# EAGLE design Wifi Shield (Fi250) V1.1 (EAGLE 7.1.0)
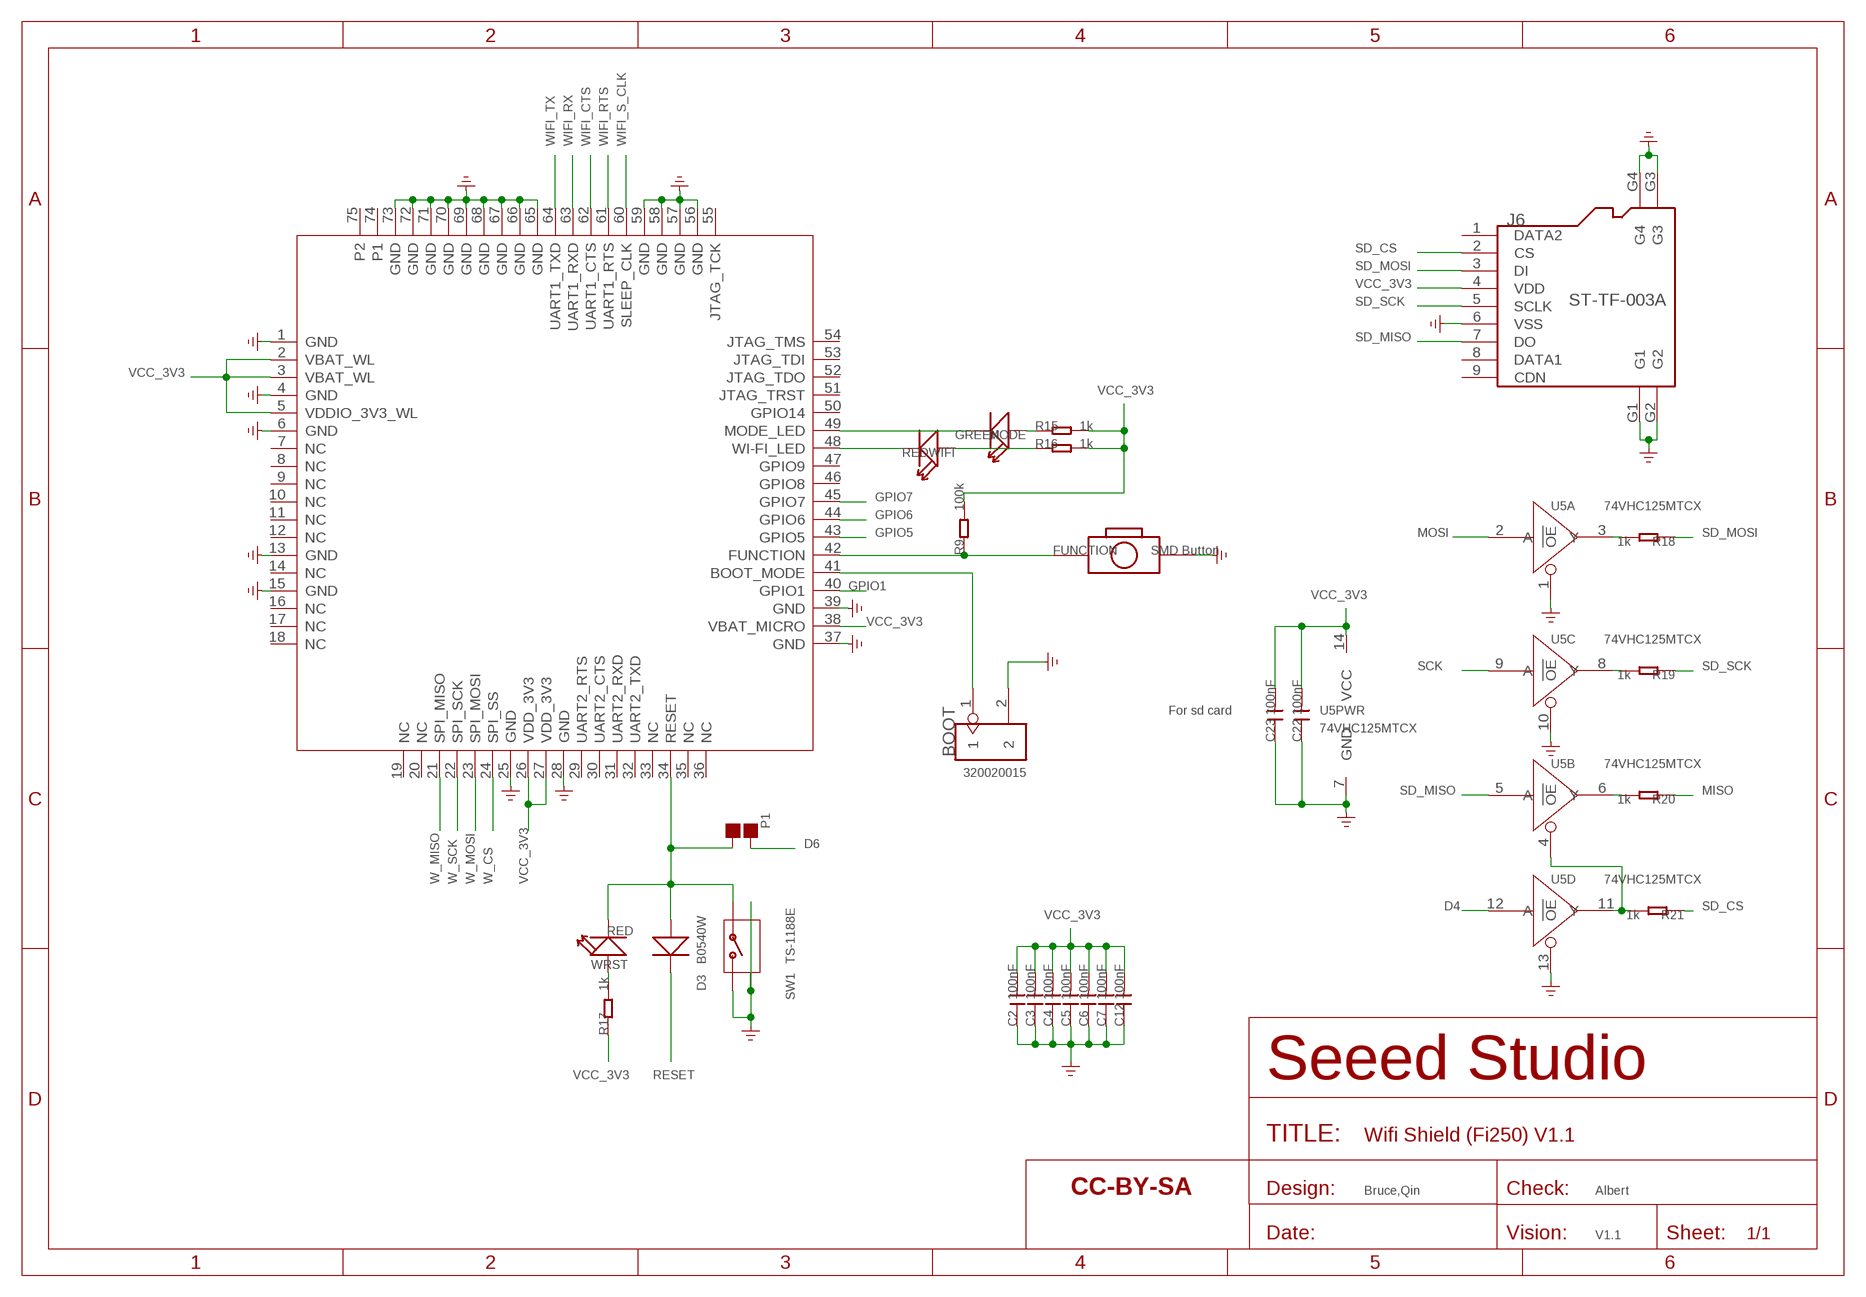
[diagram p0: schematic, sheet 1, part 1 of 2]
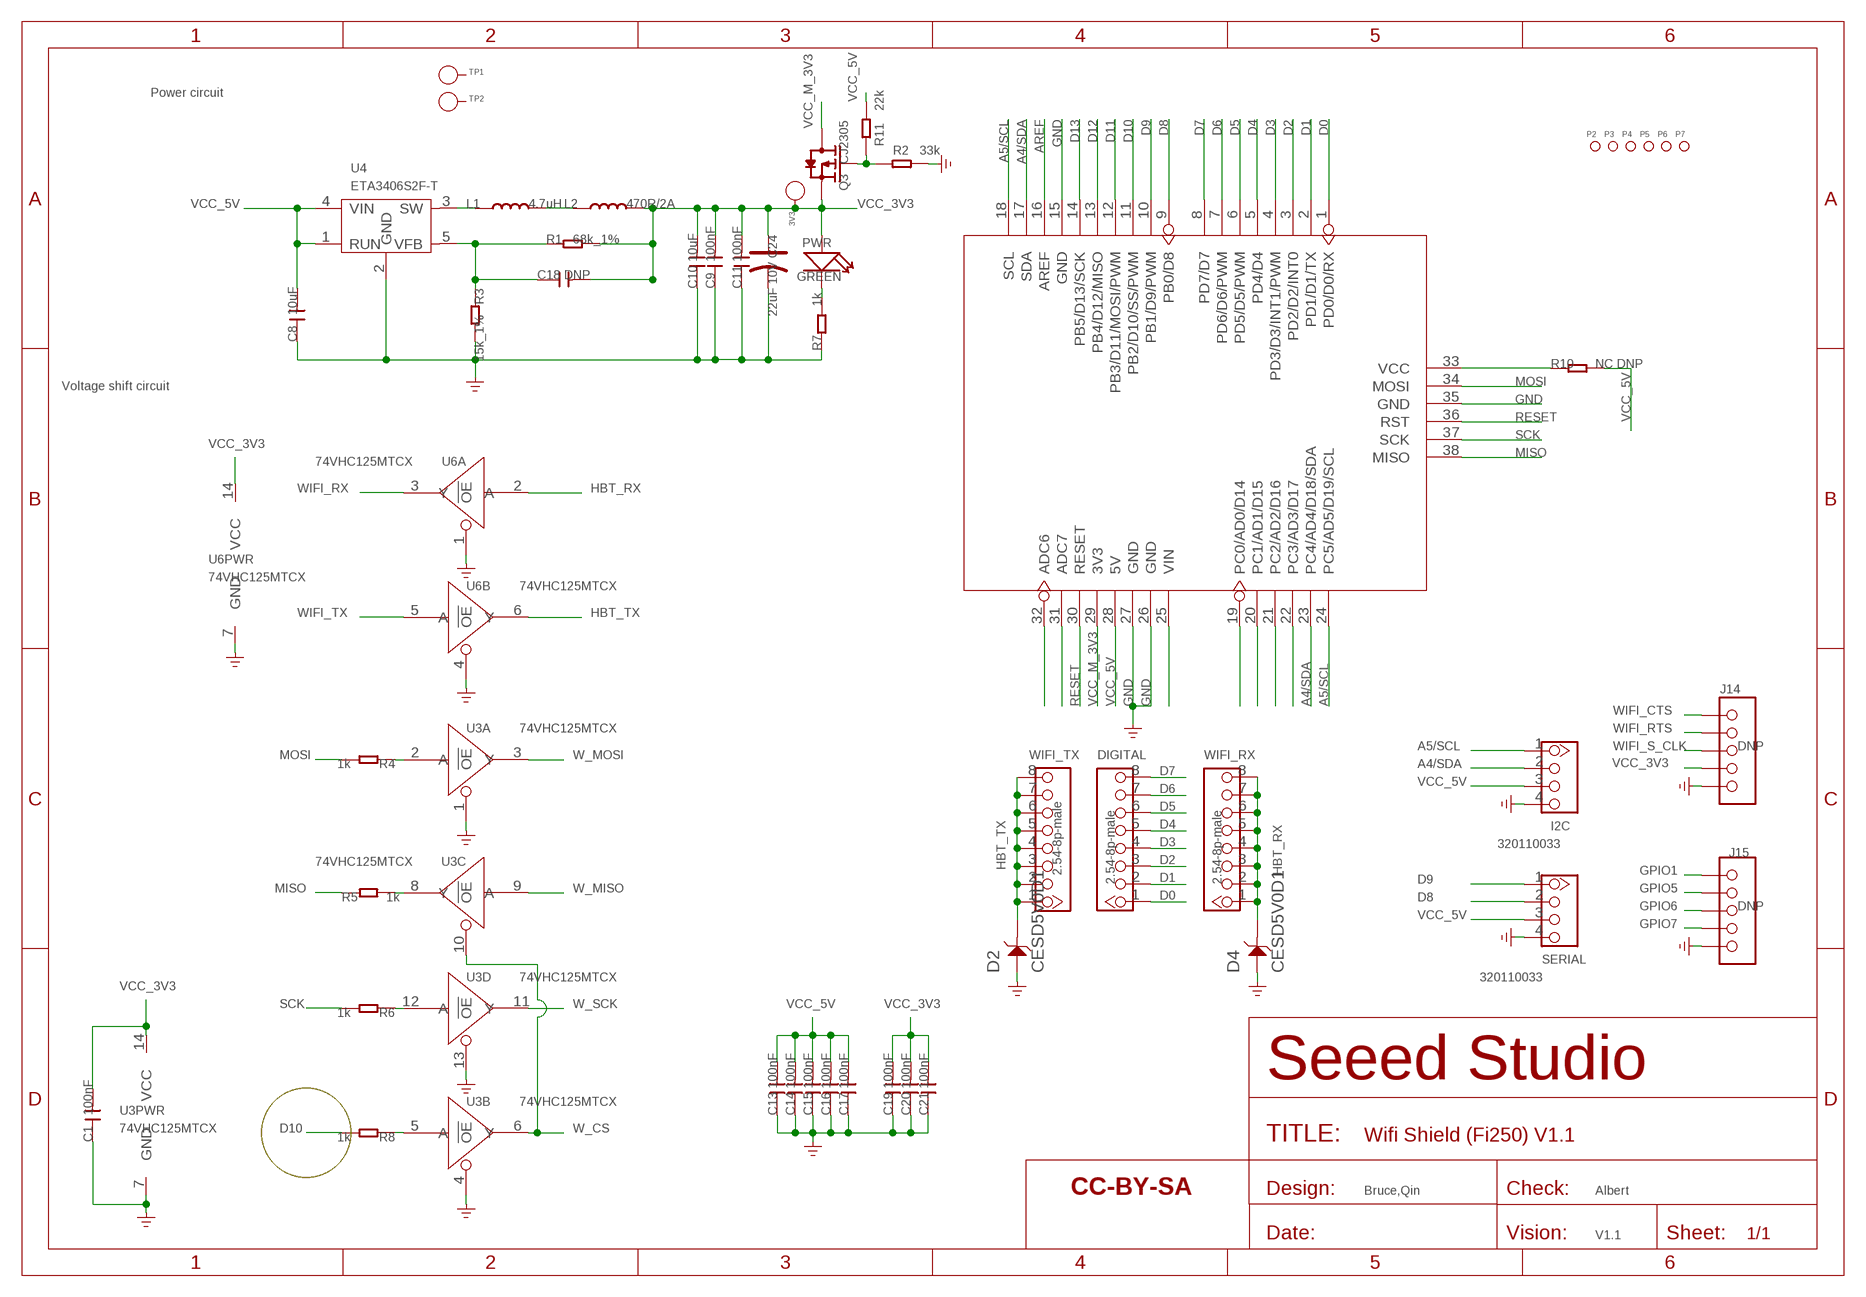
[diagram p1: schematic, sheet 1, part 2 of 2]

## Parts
3V3  PAD-TEST-POINT'4545'  [TP_4545]
BOOT  320020015  HEADER-2P-65/35MIL  [2P-2.54-65/35MIL]
C1  100nF  C-0603  [C0603]
C2  100nF  C-0603  [C0603]
C3  100nF  C-0603  [C0603]
C4  100nF  C-0603  [C0603]
C5  100nF  C-0603  [C0603]
C6  100nF  C-0603  [C0603]
C7  100nF  C-0603  [C0603]
C8  10uF  C-0805  [C0805]
C9  100nF  C-0603  [C0603]
C10  10uF  C-0805  [C0805]
C11  100nF  C-0603  [C0603]
C12  100nF  C-0603  [C0603]
C13  100nF  C-0603  [C0603]
C14  100nF  C-0603  [C0603]
C15  100nF  C-0603  [C0603]
C16  100nF  C-0603  [C0603]
C17  100nF  C-0603  [C0603]
C18  DNP  C-0603  [C0603]
C19  100nF  C-0603  [C0603]
C20  100nF  C-0603  [C0603]
C21  100nF  C-0603  [C0603]
C22  100nF  C-0603  [C0603]
C23  100nF  C-0603  [C0603]
C24  22uF 10V  CAP-AVX-A  [AVX-A]
D2  CESD5V0D1  D-ESD-2P'CESD5V0D1'  [SOD123-2.7X1.6]
D3  B0540W  D'1206'  [SOD123]
D4  CESD5V0D1  D-ESD-2P'CESD5V0D1'  [SOD123-2.7X1.6]
DIGITAL  2.54-8p-male  HEADER-8P-2.54  [8P-2.54]
FUNCTION  SMD Button  BUTTON-2P-SMD  [2P-SMD-6.1X3.81]
I2C  320110033  TWIG-4P-2.0-2.0  [4P-2.0]
J6  ST-TF-003A  HOLDER-MICROSD-9P  [9P-SMD-W/-RING]
J14  DNP  HEADER-5P-2.54  [5P-2.54]
J15  DNP  HEADER-5P-2.54  [5P-2.54]
L1  4.7uH  LSPD3D16-4R7M  [L0420]
L2  470R/2A  L'0805'  [L0805]
MODE  GREEN  LED'0603'  [LED-0603]
P1  DNP  PAD-JUMPER-2P  [2P-SMD-1.78X1.27]
P2  PAD-MARK  [ROUND-MARK-1.0]
P3  PAD-MARK  [ROUND-MARK-1.0]
P4  PAD-MARK  [ROUND-MARK-1.0]
P5  PAD-MARK  [ROUND-MARK-1.0]
P6  PAD-MARK  [ROUND-MARK-1.0]
P7  PAD-MARK  [ROUND-MARK-1.0]
PWR  GREEN  LED'0603'  [LED-0603]
Q3  CJ2305  MOSFET-P'SI2323CDS/SI2305DS<BR>'  [SOT23]
R1  68k_1%  R-0603  [R0603]
R2  33k  R-0603  [R0603]
R3  15k_1%  R-0603  [R0603]
R4  1k  R-0603  [R0603]
R5  1k  R-0603  [R0603]
R6  1k  R-0603  [R0603]
R7  1k  R-0603  [R0603]
R8  1k  R-0603  [R0603]
R9  100k  R-0603  [R0603]
R10  NC DNP  R-0603  [R0603]
R11  22k  R-0603  [R0603]
R15  1k  R-0603  [R0603]
R16  1k  R-0603  [R0603]
R17  1k  R-0603  [R0603]
R18  1k  R-0603  [R0603]
R19  1k  R-0603  [R0603]
R20  1k  R-0603  [R0603]
R21  1k  R-0603  [R0603]
SERIAL  320110033  TWIG-4P-2.0-2.0  [4P-2.0]
SW1  TS-1188E  BUTTON-4P-REINFORCE'TS-1188E'  [4P-SMD-7X3.5X3.5H]
TP1  PAD-TEST-POINT'4545'  [TP_4545]
TP2  PAD-TEST-POINT'4545'  [TP_4545]
U1  WIZFI250  [73P-28X20MM]
U2  206000005  ARDUINO-38P'WITH-SILK'  [ARDUINO-DIM-WITH-SILK]
U3  74VHC125MTCX  74VHCT125PW  [TSSOP14]
U4  ETA3406S2F-T  TD6810'TSOT23-5'  [SOT23-5]
U5  74VHC125MTCX  74VHC125PW  [TSSOP14]
U6  74VHC125MTCX  74VHC125PW  [TSSOP14]
U$1  SEEEDSTUDIO-OPEN-SCH-FRAME  [SEEEDSTUDIO-PCB-FRAME]
U$2  SEEEDSTUDIO-OPEN-SCH-FRAME  [SEEEDSTUDIO-PCB-FRAME]
WIFI  RED  LED'0603'  [LED-0603]
WIFI_RX  2.54-8p-male  HEADER-8P-2.54  [8P-2.54]
WIFI_TX  2.54-8p-male  HEADER-8P-2.54  [8P-2.54]
WRST  RED  LED'0603'  [LED-0603]

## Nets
A4/SDA: I2C.2 U2.17(SDA) U2.23(PC4/AD4/D18/SDA)
A5/SCL: I2C.1 U2.18(SCL) U2.24(PC5/AD5/D19/SCL)
AREF: U2.16(AREF)
D0: DIGITAL.1 U2.1(PD0/D0/RX)
D1: DIGITAL.2 U2.2(PD1/D1/TX)
D2: DIGITAL.3 U2.3(PD2/D2/INT0)
D3: DIGITAL.4 U2.4(PD3/D3/INT1/PWM)
D4: DIGITAL.5 U2.5(PD4/D4) U5.12(D:A)
D5: DIGITAL.6 U2.6(PD5/D5/PWM)
D6: DIGITAL.7 P1.2 U2.7(PD6/D6/PWM)
D7: DIGITAL.8 U2.8(PD7/D7)
D8: SERIAL.2 U2.9(PB0/D8)
D9: SERIAL.1 U2.10(PB1/D9/PWM)
D10: R8.2 U2.11(PB2/D10/SS/PWM)
D11: U2.12(PB3/D11/MOSI/PWM)
D12: U2.13(PB4/D12/MISO)
D13: U2.14(PB5/D13/SCK)
GND: BOOT.2 C1.1 C2.1 C3.1 C4.1 C5.1 C6.1 C7.1 C8.1 C9.1 C10.1 C11.1 C12.1 C13.1 C14.1 C15.1 C16.1 C17.1 C19.1 C20.1 C21.1 C22.1 C23.1 C24.- D2.1 D4.1 FUNCTION.P$2 I2C.4 J6.6(VSS) J6.G1 J6.G2 J6.G3 J6.G4 J14.5 J15.5 R2.1 R3.2 R7.1 SERIAL.4 SW1.2 SW1.S1 SW1.S2 U1.1(GND) U1.4(GND) U1.6(GND) U1.13(GND) U1.15(GND) U1.25(GND) U1.28(GND) U1.37(GND) U1.39(GND) U1.56(GND) U1.57(GND) U1.58(GND) U1.59(GND) U1.65(GND) U1.66(GND) U1.67(GND) U1.68(GND) U1.69(GND) U1.70(GND) U1.71(GND) U1.72(GND) U1.73(GND) U2.15(GND) U2.26(GND) U2.27(GND) U2.35(GND) U3.1(A:!OE) U3.4(B:!OE) U3.7(PWR:GND) U3.13(D:!OE) U4.2(GND) U5.1(A:!OE) U5.7(PWR:GND) U5.10(C:!OE) U5.13(D:!OE) U6.1(A:!OE) U6.4(B:!OE) U6.7(PWR:GND)
GPIO1: J15.1 U1.40(GPIO1)
GPIO5: J15.2 U1.43(GPIO5)
GPIO6: J15.3 U1.44(GPIO6)
GPIO7: J15.4 U1.45(GPIO7)
HBT_RX: D4.2 U6.2(A:A) WIFI_RX.1 WIFI_RX.2 WIFI_RX.3 WIFI_RX.4 WIFI_RX.5 WIFI_RX.6 WIFI_RX.7 WIFI_RX.8
HBT_TX: D2.2 U6.6(B:Y) WIFI_TX.1 WIFI_TX.2 WIFI_TX.3 WIFI_TX.4 WIFI_TX.5 WIFI_TX.6 WIFI_TX.7 WIFI_TX.8
MISO: R5.1 R20.1 U2.38(MISO)
MOSI: R4.2 U2.34(MOSI) U5.2(A:A)
N$1: R10.1 U2.33(VCC)
N$2: BOOT.1 U1.41(BOOT_MODE)
N$3: R4.1 U3.2(A:A)
N$4: R6.1 U3.12(D:A)
N$6: R5.2 U3.8(C:Y)
N$7: FUNCTION.1 R9.1 U1.42(FUNCTION)
N$8: L1.1 U4.3(SW)
N$9: R17.2 WRST.+
N$10: L1.2 L2.1
N$12: MODE.- U1.49(MODE_LED)
N$13: U1.48(WI-FI_LED) WIFI.-
N$14: U2.32(ADC6)
N$15: R16.1 WIFI.+
N$18: MODE.+ R15.1
N$20: D3.+ P1.1 SW1.1 U1.34(RESET) WRST.-
N$23: Q3.1(G) R2.2 R11.2
N$24: R18.2 U5.3(A:Y)
N$25: U2.31(ADC7)
N$26: PWR.- R7.2
N$27: R8.1 U3.5(B:A)
N$28: R19.2 U5.8(C:Y)
N$29: R20.2 U5.6(B:Y)
N$30: R21.2 U5.4(B:!OE) U5.11(D:Y)
N$36: U2.25(VIN)
N$37: U2.19(PC0/AD0/D14)
N$38: U2.20(PC1/AD1/D15)
N$39: C18.1 R1.1 R3.1 U4.5(VFB)
N$40: U2.21(PC2/AD2/D16)
N$41: U2.22(PC3/AD3/D17)
RESET: D3.- U2.30(RESET) U2.36(RST)
SCK: R6.2 U2.37(SCK) U5.9(C:A)
SD_CS: J6.2(CS) R21.1
SD_MISO: J6.7(DO) U5.5(B:A)
SD_MOSI: J6.3(DI) R18.1
SD_SCK: J6.5(SCLK) R19.1
VCC_3V3: 3V3.T C1.2 C2.2 C3.2 C4.2 C5.2 C6.2 C7.2 C9.2 C10.2 C11.2 C12.2 C18.2 C19.2 C20.2 C21.2 C22.2 C23.2 C24.+ J6.4(VDD) J14.4 L2.2 PWR.+ Q3.2(S) R1.2 R9.2 R15.2 R16.2 R17.1 U1.2(VBAT_WL) U1.3(VBAT_WL) U1.5(VDDIO_3V3_WL) U1.26(VDD_3V3) U1.27(VDD_3V3) U1.38(VBAT_MICRO) U3.14(PWR:VCC) U5.14(PWR:VCC) U6.14(PWR:VCC)
VCC_5V: C8.2 C13.2 C14.2 C15.2 C16.2 C17.2 I2C.3 R10.2 R11.1 SERIAL.3 U2.28(5V) U4.1(RUN) U4.4(VIN)
VCC_M_3V3: Q3.3(D) U2.29(3V3)
W_CS: U1.24(SPI_SS) U3.6(B:Y) U3.10(C:!OE)
W_MISO: U1.21(SPI_MISO) U3.9(C:A)
W_MOSI: U1.23(SPI_MOSI) U3.3(A:Y)
W_SCK: U1.22(SPI_SCK) U3.11(D:Y)
WIFI_CTS: J14.1 U1.62(UART1_CTS)
WIFI_RTS: J14.2 U1.61(UART1_RTS)
WIFI_RX: U1.63(UART1_RXD) U6.3(A:Y)
WIFI_S_CLK: J14.3 U1.60(SLEEP_CLK)
WIFI_TX: U1.64(UART1_TXD) U6.5(B:A)
Unconnected: J6.1(DATA2) J6.8(DATA1) J6.9(CDN) TP1.T TP2.T U1.7(NC) U1.8(NC) U1.9(NC) U1.10(NC) U1.11(NC) U1.12(NC) U1.14(NC) U1.16(NC) U1.17(NC) U1.18(NC) U1.19(NC) U1.20(NC) U1.29(UART2_RTS) U1.30(UART2_CTS) U1.31(UART2_RXD) U1.32(UART2_TXD) U1.33(NC) U1.35(NC) U1.36(NC) U1.46(GPIO8) U1.47(GPIO9) U1.50(GPIO14) U1.51(JTAG_TRST) U1.52(JTAG_TDO) U1.53(JTAG_TDI) U1.54(JTAG_TMS) U1.55(JTAG_TCK) U1.74(P1) U1.75(P2) U6.8(C:Y) U6.9(C:A) U6.10(C:!OE) U6.11(D:Y) U6.12(D:A) U6.13(D:!OE)

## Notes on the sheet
- Power circuit
- Voltage shift circuit
- For sd card
- Bruce,Qin | Albert | Bruce,Qin | Albert
- V1.1 | V1.1

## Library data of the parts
3V3 TP1 TP2 = Discrete:PAD-TEST-POINT; PARTNO: DNP
BOOT = Connector :HEADER-2P
C1-C23 = Discrete:C*: Ceramic Capacitors
C24 = Discrete:CAP*: Electrolytic Capacitors,Tantalum Capacitors and Super Capacitors
D2 D4 = Discrete:D-ESD-2P: Diodes for Protectiong against ESD
D3 = Discrete:D*
DIGITAL WIFI_RX WIFI_TX = Connector:HEADER-8P
FUNCTION = Discrete:BUTTON-2P
I2C SERIAL = Connector:TWIG-4P-2.0
J6 = Connector :HOLDER-MICROSD-9P
J14 J15 = Connector:HEADER-5P
L1 = template:L
L2 = Discrete:L*
MODE PWR WIFI WRST = Discrete:LED*
P1 = Discrete:PAD-JUMPER-2P; PARTNO: DNP
P2-P7 = Discrete:PAD-MARK; PARTNO: DNP
Q3 = Discrete:MOSFET-P
R1-R11 R15-R21 = Discrete:R*
SW1 = Discrete:BUTTON-4P-REINFORCE: TS-1188E http://www.best-dz.com/?thread-374-2.html
U1 = template:WIZFI250: The WizFi250 provides for the highest-level integration, featuring 802.11b/g and 802.11n. It includes a 2.4 GHz WLAN CMOS power amplifier (PA) that meets the output power requirements of most handheld systems.
U2 = moudle-new:ARDUINO-38P
U3 U5 U6 = IC:74V*125: Quad Buffer/Line Driver;3-state
U4 = template:TD6810: 1.5MHz 800mA Synchronous Step-Down Regulator Dropout http://www.techcodeok.com/download/TD6810.pdf
U$1 U$2 = moudle-new:SEEEDSTUDIO-OPEN-SCH-FRAME

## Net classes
0 default: width 0.152 mm, drill 0.305 mm, clearance 0.152 mm

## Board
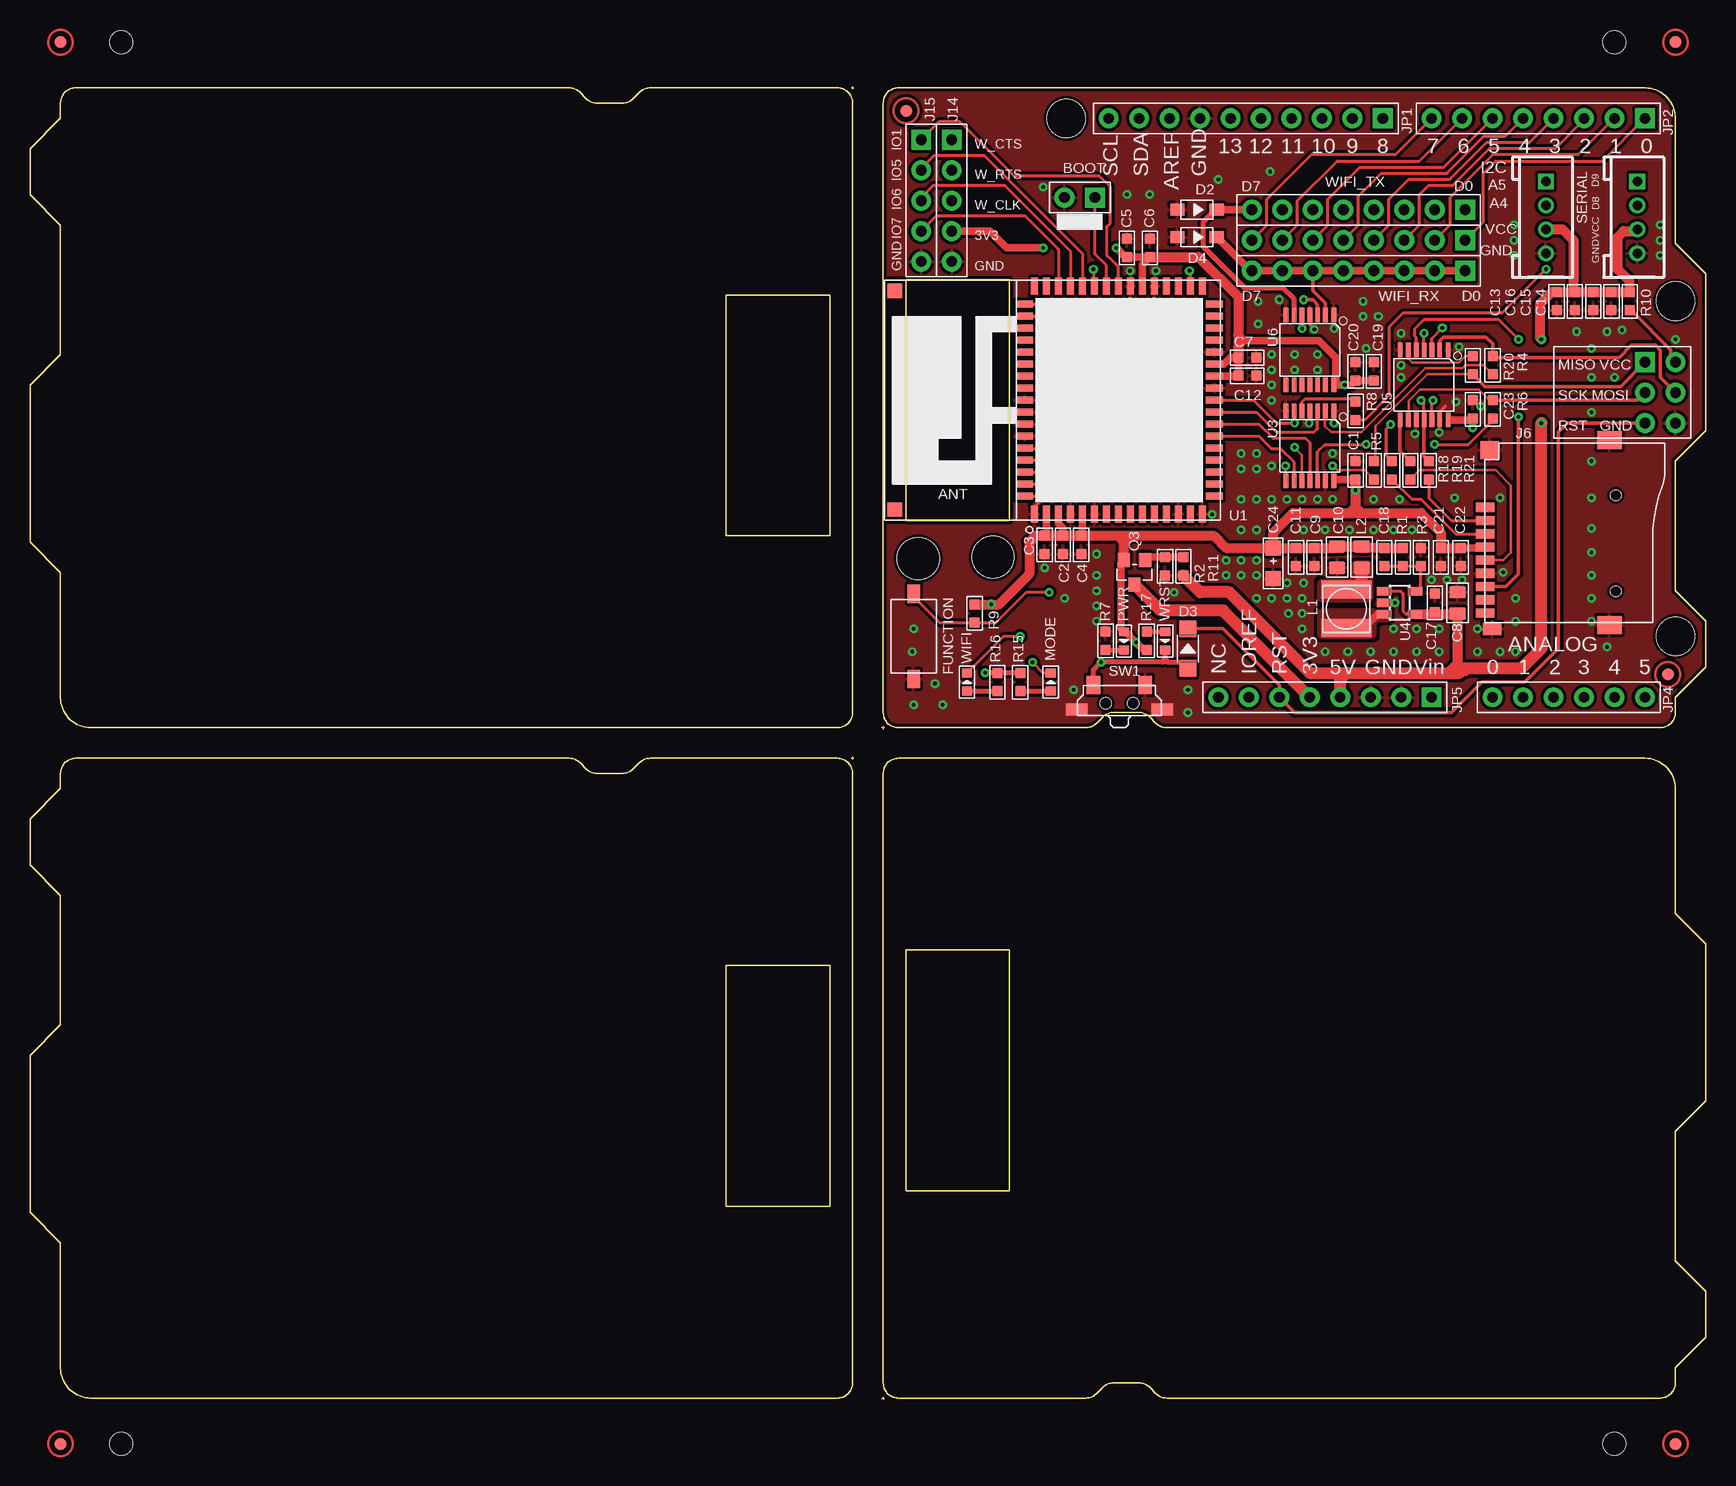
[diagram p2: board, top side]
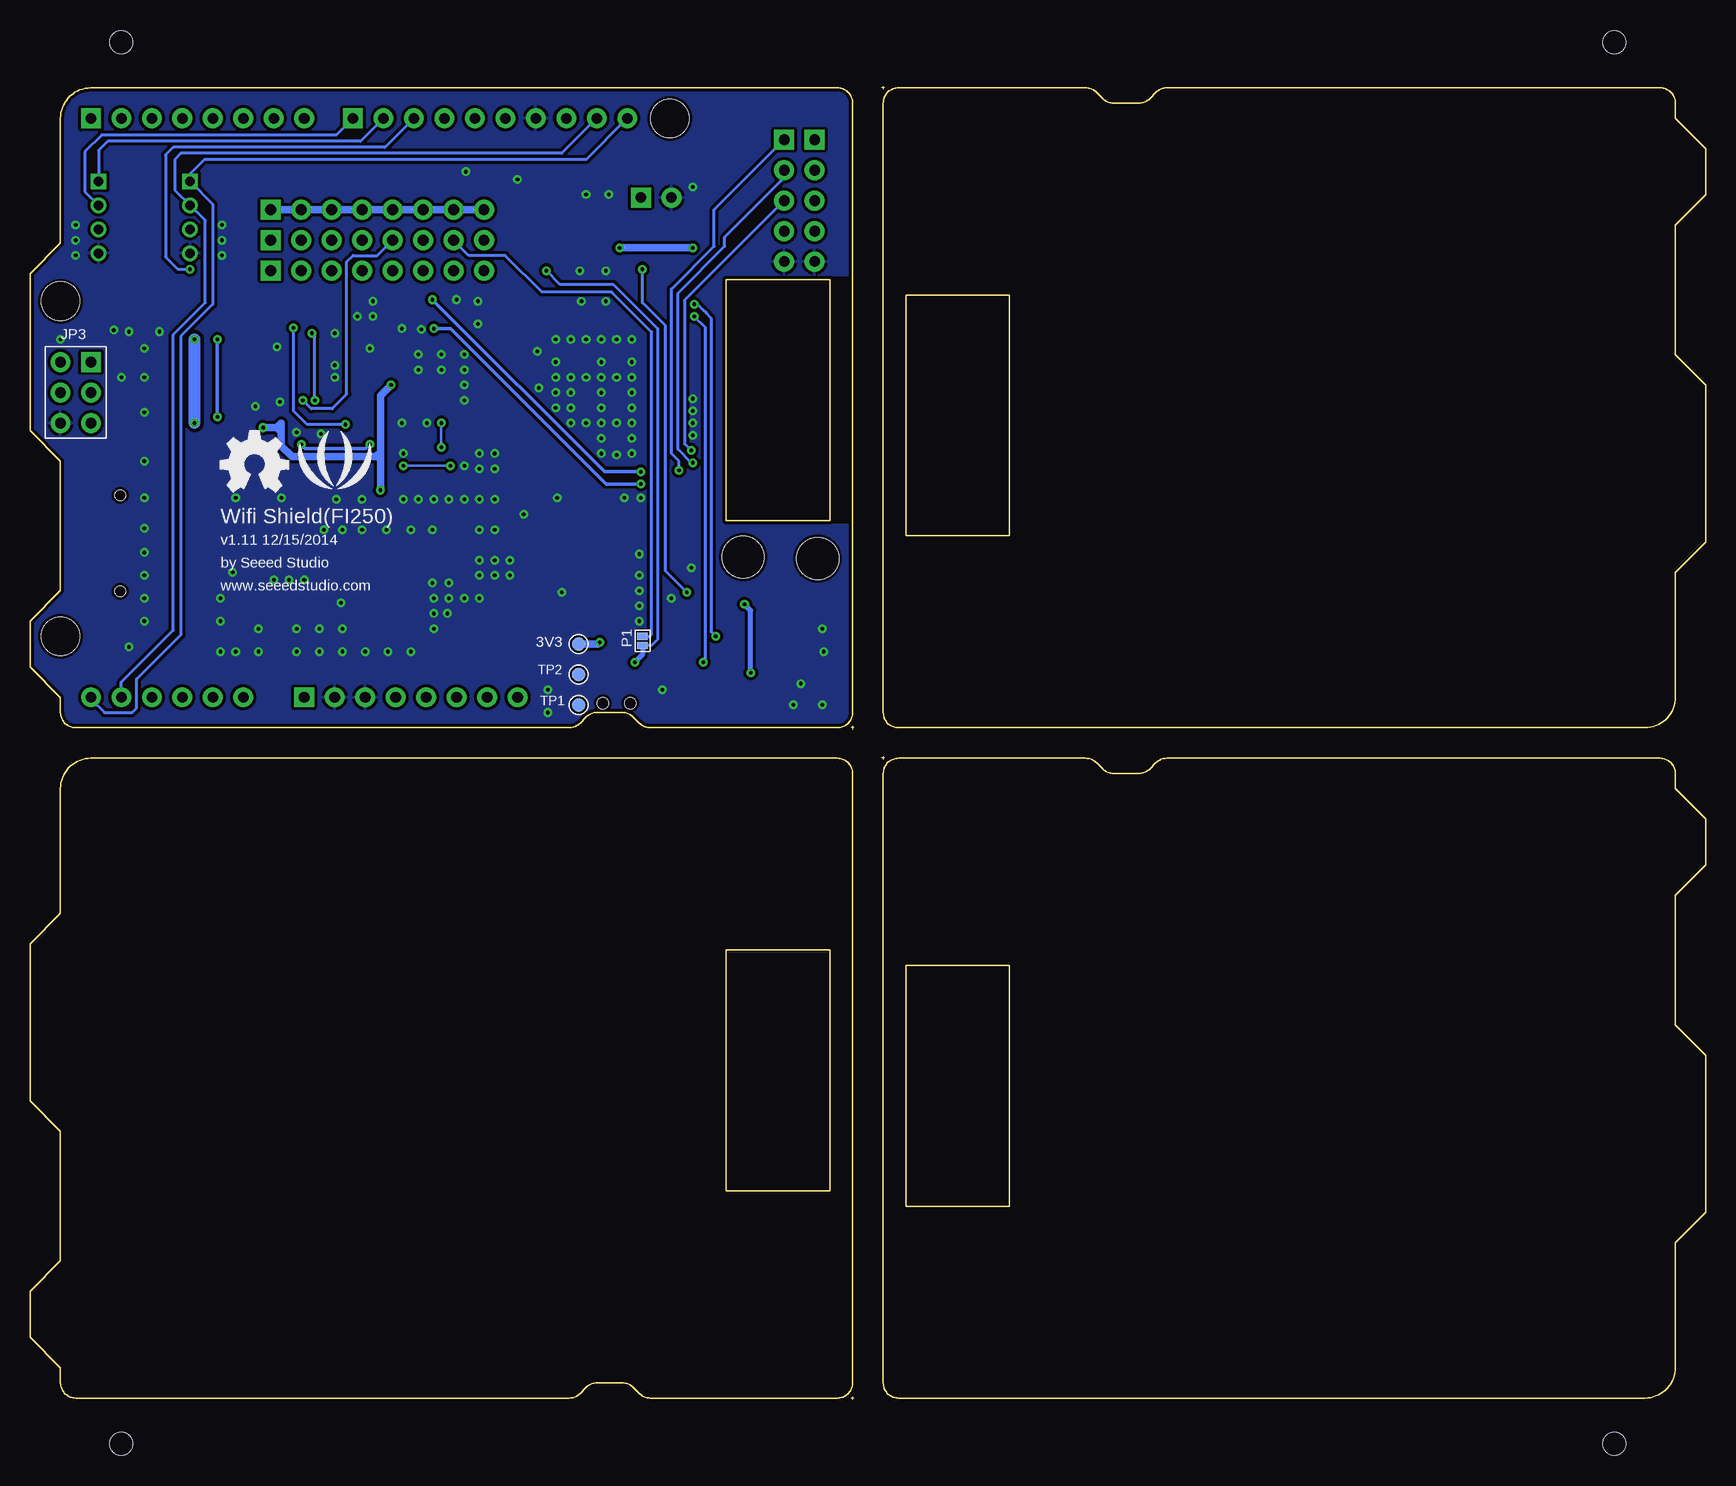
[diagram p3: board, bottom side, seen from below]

Size 139.7 x 109.47 mm. Coordinates in mm from the lower left corner, seen from the top.
Outline: 120 segments
Copper layers (1*16): Top 0.035mm / dielectric 1.5mm / Bottom 0.035mm
Design rules "default *": minimum track width 6mil, minimum drill 12mil, track to track 8mil, track to pad 8mil, pad to pad 8mil, via to via 8mil, smd to smd 0mil, copper to edge 10mil, drill to drill 8mil, minimum pad ring 10mil, minimum via ring 8mil, stop-mask expansion 4mil, vias tented up to drill 100mil, thermal gap 10mil
Holes 3.5 mm at 80.26,70.23 74.04,70.1
Holes 3.2 mm at 86.36,106.81 137.16,63.63 137.16,91.57
Holes 1.91 mm at 7.62,113.16 132.08,113.16 132.08,-3.68 7.62,-3.68
tRestrict: area 82.7,82.8 to 83.3,82.9; area 82.7,81.8 to 83.3,81.9; area 82.7,80.8 to 83.3,80.9

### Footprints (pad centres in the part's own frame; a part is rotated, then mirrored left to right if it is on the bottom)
TP_4545 = smd 1.143 x 1.143: T 0,0
2P-2.54-65/35MIL = drill 0.889 pad 1.651 square: 1 0,1.27 | drill 0.889 pad 1.651: 2 0,-1.27
C0603 = smd 0.889 x 0.889: 1 -0.762,0; 2 0.762,0
C0805 = smd 1.016 x 1.397: 1 -0.889,0; 2 0.889,0
AVX-A = smd 1.27 x 1.27: + -1.27,0; - 1.27,0
SOD123-2.7X1.6 = smd 1.2 x 1.02: 1 -1.635,0; 2 1.635,0
SOD123 = smd 1.397 x 1.397: + -1.651,0; - 1.651,0
8P-2.54 = drill 0.889 pad 1.651 square: 1 0,8.89 | drill 0.889 pad 1.651: 2 0,6.35; 3 0,3.81; 4 0,1.27; 5 0,-1.27; 6 0,-3.81; 7 0,-6.35; 8 0,-8.89
2P-SMD-6.1X3.81 = smd 1.524 x 1.016: 1 -3.556,0; P$2 3.556,0
4P-2.0 = drill 0.8 pad 1.27 square: 1 -3,0 | drill 0.8 pad 1.27: 2 -1,0; 3 1,0; 4 3,0
9P-SMD-W/-RING = smd 1.524 x 0.762: 1 0,4.4; 2 0,3.3; 3 0,2.2; 4 0,1.1; 5 0,0; 6 0,-1.1; 7 0,-2.2; 8 0,-3.3; 9 0,-4.4 | smd 1.524 x 1.016: G1 0.6,-5.746 | smd 2.032 x 1.524: G2 10.373,-5.4; G3 10.373,10 | smd 1.524 x 1.524: G4 0.392,9.181 | hole 0.889: 10.9,-2.6; 10.9,5.4
5P-2.54 = drill 0.889 pad 1.651 square: 1 0,5.08 | drill 0.889 pad 1.651: 2 0,2.54; 3 0,0; 4 0,-2.54; 5 0,-5.08
L0420 = smd 1.5 x 4.2: 1 -1.6,0; 2 1.6,0
L0805 = smd 1.016 x 1.397: 1 -0.889,0; 2 0.889,0
LED-0603 = smd 0.762 x 0.889: + -0.762,0; - 0.762,0
2P-SMD-1.78X1.27 = smd 0.889 x 0.61: 1 0,0.381; 2 0,-0.381
ROUND-MARK-1.0 = smd 1.016 x 1.016: P$1 0,0
SOT23 = smd 1.016 x 1.143: 1 -0.889,-1.016; 2 0.889,-1.016; 3 0,1.016
R0603 = smd 0.889 x 0.889: 1 -0.762,0; 2 0.762,0
4P-SMD-7X3.5X3.5H = smd 1.143 x 1.524: 1 -2.159,1.524; 2 2.159,1.524 | smd 1.778 x 1.016: S1 -3.556,-0.508; S2 3.556,-0.508 | hole 0.95: -1.15,0; 1.15,0
73P-28X20MM = smd 0.6 x 1.4: 1 -1.5,-9.5; 2 -0.5,-9.5; 3 0.5,-9.5; 4 1.5,-9.5; 5 2.5,-9.5; 6 3.5,-9.5; 7 4.5,-9.5; 8 5.5,-9.5; 9 6.5,-9.5; 10 7.5,-9.5; 11 8.5,-9.5; 12 9.5,-9.5; 13 10.5,-9.5; 14 11.5,-9.5; 15 12.5,-9.5; 33 12.5,9.5; 34 11.5,9.5; 35 10.5,9.5; 36 9.5,9.5; 37 8.5,9.5; 38 7.5,9.5; 39 6.5,9.5; 40 5.5,9.5; 41 4.5,9.5; 42 3.5,9.5; 43 2.5,9.5; 44 1.5,9.5; 45 0.5,9.5; 46 -0.5,9.5; 47 -1.5,9.5 | smd 1.4 x 0.6: 16 13.5,-8; 17 13.5,-7; 18 13.5,-6; 19 13.5,-5; 20 13.5,-4; 21 13.5,-3; 22 13.5,-2; 23 13.5,-1; 24 13.5,0; 25 13.5,1; 26 13.5,2; 27 13.5,3; 28 13.5,4; 29 13.5,5; 30 13.5,6; 31 13.5,7; 32 13.5,8; 48 -2.3,8; 49 -2.3,7; 50 -2.3,6; 51 -2.3,5; 52 -2.3,4; 53 -2.3,3; 54 -2.3,2; 55 -2.3,1; 56 -2.3,0; 57 -2.3,-1; 58 -2.3,-2; 59 -2.3,-3; 60 -2.3,-4; 61 -2.3,-5; 62 -2.3,-6; 63 -2.3,-7; 64 -2.3,-8 | smd 1.2 x 1.2: 65 2.5,-3.5; 66 5.5,-3.5; 67 8.5,-3.5; 68 2.5,0; 69 5.5,0; 70 8.5,0; 71 2.5,3.5; 72 5.5,3.5; 73 8.5,3.5; 74 -13.12,9.12; 75 -13.12,-9.12
ARDUINO-DIM-WITH-SILK = drill 0.889 pad 1.651 square: 1 63.5,50.8; 9 41.656,50.8; 25 45.72,2.54; 38 63.5,30.48 | drill 0.889 pad 1.651: 2 60.96,50.8; 3 58.42,50.8; 4 55.88,50.8; 5 53.34,50.8; 6 50.8,50.8; 7 48.26,50.8; 8 45.72,50.8; 10 39.116,50.8; 11 36.576,50.8; 12 34.036,50.8; 13 31.496,50.8; 14 28.956,50.8; 15 26.416,50.8; 16 23.876,50.8; 17 21.336,50.8; 18 18.796,50.8; 19 50.8,2.54; 20 53.34,2.54; 21 55.88,2.54; 22 58.42,2.54; 23 60.96,2.54; 24 63.5,2.54; 26 43.18,2.54; 27 40.64,2.54; 28 38.1,2.54; 29 35.56,2.54; 30 33.02,2.54; 31 30.48,2.54; 32 27.94,2.54; 33 66.04,30.48; 34 66.04,27.94; 35 66.04,25.4; 36 63.5,25.4; 37 63.5,27.94 | hole 3.2: 15.24,50.8; 66.04,35.56; 66.04,7.62
TSSOP14 = smd 0.4 x 1.2: 1 -2,-2.925; 2 -1.3,-2.925; 3 -0.65,-2.925; 4 0,-2.925; 5 0.65,-2.925; 6 1.3,-2.925; 7 2,-2.925; 8 2,2.925; 9 1.3,2.925; 10 0.65,2.925; 11 0,2.925; 12 -0.65,2.925; 13 -1.3,2.925; 14 -2,2.925
SOT23-5 = smd 0.69 x 1.2: 1 -0.95,-1.3; 2 0,-1.3; 3 0.95,-1.3; 4 0.95,1.3; 5 -0.95,1.3

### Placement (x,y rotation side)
3V3  93.98,62.99 0 bottom
BOOT  87.5,100.2 270 top
C1  110.49,77.47 270 top
C2  86.11,71.25 90 top
C3  84.58,71.25 90 top
C4  87.63,71.25 90 top
C5  91.44,96.01 270 top
C6  93.34,96.01 270 top
C7  101.47,86.87 180 top
C8  119,66.42 270 top
C9  107.06,70.23 90 top
C10  108.97,70.23 90 top
C11  105.54,70.23 90 top
C12  101.47,85.34 180 top
C13  127.25,91.57 90 top
C14  131.83,91.57 90 top
C15  130.3,91.57 90 top
C16  128.78,91.57 90 top
C17  117.09,66.42 270 top
C18  112.9,70.23 90 top
C19  112.01,85.72 270 top
C20  110.49,85.72 270 top
C21  117.6,70.23 90 top
C22  119.25,70.23 90 top
C23  120.27,82.55 270 top
C24  103.63,69.72 270 top
D2  97.28,99.19 0 top
D3  96.52,62.61 90 top
D4  97.28,96.9 0 top
DIGITAL  110.74,96.65 270 top
FUNCTION  73.66,63.63 270 top
I2C  126.37,98.55 270 top
J6  121.28,69.98 0 top
J14  76.84,99.95 0 top
J15  74.3,99.95 0 top
L1  109.73,65.91 90 top
L2  111,70.23 90 top
MODE  85.09,59.82 90 top
P1  88.65,63.25 180 bottom
P2  73.03,107.44 0 top
P3  136.53,60.45 0 top
P4  not placed on the board
P5  not placed on the board
P6  not placed on the board
P7  not placed on the board
PWR  91.19,63.25 270 top
Q3  92.08,68.96 180 top
R1  114.43,70.23 90 top
R2  94.62,69.47 90 top
R3  115.95,70.23 90 top
R4  121.92,86.23 90 top
R5  112.01,77.47 270 top
R6  121.92,82.55 90 top
R7  89.66,63.25 270 top
R8  110.49,82.42 270 top
R9  78.74,65.53 90 top
R10  133.35,91.57 90 top
R11  96.14,69.47 90 top
R15  82.55,59.82 90 top
R16  80.65,59.82 90 top
R17  93.09,63.25 90 top
R18  113.54,77.47 90 top
R19  115.06,77.47 90 top
R20  120.27,86.23 90 top
R21  116.59,77.47 90 top
SERIAL  133.99,98.55 270 top
SW1  90.81,58.04 0 top
TP1  93.98,57.91 180 bottom
TP2  93.98,60.45 0 bottom
U1  85.22,83.31 0 top
U2  71.12,56.01 0 top
U3  106.68,79.5 180 top
U4  114.17,66.42 270 top
U5  116.21,84.58 180 top
U6  106.68,87.5 180 top
U$1  not placed on the board
U$2  not placed on the board
U$23  [OSHW_FILLX200_NOTEXT]  123.83,75.69 0 bottom
U$24  [LOGO_SILK]  114.3,77.6 0 bottom
WIFI  78.11,59.82 90 top
WIFI_RX  110.74,94.11 270 top
WIFI_TX  110.74,99.19 270 top
WRST  94.62,63.25 270 top

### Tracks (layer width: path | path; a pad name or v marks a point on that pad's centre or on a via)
A4/SDA
  Bottom 0.254: U2.23 132.08,59.82 127.76,64.13 127.76,88.77 125.09,91.44 125.09,98.31 126.35,99.57 I2C.2 127.64,100.82 127.64,103.38 127.13,103.89 95.38,103.89 U2.17
A5/SCL
  Bottom 0.254: U2.24 134.62,58.42 133.48,57.28 131.19,57.28 130.81,57.66 130.81,60.07 127.13,63.75 127.13,88.65 124.46,91.31 124.46,99.65 I2C.1 126.37,102.19 125.17,103.38 93.34,103.38 U2.18
D0
  Top 0.254: DIGITAL.1 121.16,98.17 121.16,102.23 122.18,103.25 131.06,103.25 U2.1
D1
  Top 0.254: DIGITAL.2 118.36,97.92 118.36,100.2 121.92,103.76 129.03,103.76 U2.2
D2
  Top 0.254: DIGITAL.3 115.82,97.92 115.82,100.46 116.59,101.22 118.62,101.22 121.67,104.27 127.13,104.27 129.54,106.68 U2.3
D3
  Top 0.254: DIGITAL.4 113.28,97.92 113.28,100.08 114.94,101.73 118.36,101.73 121.41,104.78 124.97,104.78 U2.4
D4  (via drill 0.3 pad 0.64)
  Top 0.254: DIGITAL.5 110.74,97.92 110.74,100.33 112.65,102.23 118.11,102.23 121.16,105.28 122.94,105.28 U2.5 | U5.12 116.86,83.2 v116.97,83.31
  Bottom 0.254: DIGITAL.5 110.74,95.38 112.78,95.38 113.28,94.87 113.28,83.82 114.51,82.59 116.25,82.59 v116.97,83.31
D5
  Top 0.254: DIGITAL.6 108.2,97.92 108.2,100.08 110.87,102.74 117.86,102.74 U2.6
D6
  Top 0.254: DIGITAL.7 105.66,97.92 105.66,99.94 108.98,103.25 115.82,103.25 U2.7
  Bottom 0.254: P1.2 88.06,63.63 87.88,63.81 87.88,89 91.22,92.33 97.03,92.33 100.08,95.38 103.12,95.38 DIGITAL.7
D7
  Top 0.254: DIGITAL.8 103.12,97.92 103.12,100.08 106.81,103.76 113.79,103.76 U2.8
D8
  Bottom 0.254: U2.9 114.17,105.41 133.73,105.41 135.13,104.01 135.13,100.69 SERIAL.2
D9
  Bottom 0.254: SERIAL.1 133.99,104.14 133.22,104.9 112.14,104.9 U2.10
D10  (via drill 0.3 pad 0.64)
  Top 0.254: v126.37,94.23 122.68,90.55 114.43,90.55 113.28,89.41 113.28,83.69 111.25,81.66 R8.2
  Bottom 0.254: U2.11 110.11,104.39 127.76,104.39 128.4,103.76 128.4,95.25 127.38,94.23 v126.37,94.23
GND  (via drill 0.3 pad 0.64)
  Top 0.254: U3.4 106.68,81.47 v106.62,81.41
  Top 0.305: U6.4 106.68,89.66 107.06,89.28 | U1.1 83.72,74.38 84.58,75.25 88.71,75.25 v88.77,75.18 | U5.13 117.5,82.33 117.98,82.8
  other vias: 103.38,102.36 91.44,100.46 93.34,100.46 99.06,101.73 128.91,89.03 131.44,89.03 137.16,88.39 132.72,89.15 120.9,82.8 103.5,87.12 103.5,85.85 105.41,87.12 105.41,85.85 107.31,87.12 107.31,85.85 103.5,84.58 103.5,83.31 103.5,77.85 130.18,78.23 108.59,78.87 111.12,91.57 111.38,87.63 111.12,90.3 112.4,90.3 104.78,66.8 106.05,66.8 106.17,68.07 104.78,68.07 106.05,65.53 104.9,65.53 106.05,64.26 102.23,66.8 107.95,62.36 109.86,62.36 111.76,62.36 113.67,62.36 115.57,62.36 117.47,62.36 117.47,64.26 115.57,64.26 113.67,64.26 113.79,66.42 116.84,68.33 118.11,68.33 119.38,68.33 103.5,66.8 102.23,68.71 102.23,69.98 100.97,69.98 99.7,69.98 99.7,68.71 100.97,68.71 109.98,72.52 112.01,72.52 107.95,72.52 106.17,72.52 113.67,72.52 115.19,72.52 95.38,67.31 88.9,70.48 88.9,68.71 88.9,67.44 88.9,66.17 88.9,64.9 96.52,59.18 96.52,57.28 87,59.18 102.23,72.52 100.97,72.52 100.97,75.06 102.23,75.06 102.23,77.6 100.97,77.6 100.97,78.87 102.23,78.87 106.05,75.06 108.59,75.06 112.01,75.06 114.17,75.06 118.75,75.18 122.56,75.18 130.18,75.18 130.18,72.64 130.18,70.61 130.18,68.71 130.18,66.8 130.18,64.9 123.83,64.9 123.83,66.8 122.81,68.96 120.65,62.36 120.65,64.26 122.56,62.36 123.83,62.36 131.44,62.74 132.08,85.22 130.18,85.22 130.18,82.3 130.18,87.63 114.3,86.23 114.3,85.22 114.3,88.9 108.71,89.28 104.14,91.69 102.36,91.57 102.36,89.66 107.31,75.06 104.78,75.06 103.5,75.06 119.13,87.76 107.06,89.22 90.81,88.39 89.53,88.39 89.53,86.49 89.53,85.22 90.81,85.22 92.08,85.22 92.08,86.49 92.08,88.39 89.53,83.95 92.08,83.95 92.08,82.68 89.53,82.68 89.53,81.41 90.81,81.41 92.08,81.41 92.08,80.14 92.08,78.87 90.81,78.74 89.53,78.87 89.53,80.14 93.34,81.41 94.62,81.41 93.34,85.22 93.34,88.39 94.62,88.39 94.62,85.22 95.89,85.22 95.89,86.49 95.89,88.39 95.89,83.95 95.89,82.68 94.62,83.95 94.62,82.68 90.17,75.18 93.85,94.11 91.69,94.11 97.41,87.38 97.28,84.33 95.76,75.18 98.55,73.79 91.69,91.57 93.73,91.57 84.46,80.39 84.46,82.42 84.46,81.41 84.46,83.44 84.46,101.09 115.44,80.52 117.47,80.64 108.71,81.41 123.7,96.65 123.7,95.38 123.7,97.92 135.89,97.92 135.89,96.65 135.89,95.38 75.44,59.69 73.53,62.36 73.66,64.26 73.66,57.91 76.07,57.91 118.87,83.19 86.23,66.8 84.58,69.34
  pour Bottom (isolate 0.254, rank 6): 71.12,109.98 139.7,109.98 139.7,56.01 71.12,56.01 71.12,72.9 73.03,72.9 73.03,93.73 71.12,93.73
  pour Top (isolate 0.254, rank 6): 71.12,109.98 139.7,109.98 139.7,56.01 71.12,56.01 71.12,72.9 73.03,72.9 73.03,93.73 71.12,93.73
GPIO1
  Top 0.254: J15.1 75.82,106.55 77.47,106.55 82.04,101.98 89.15,101.98 90.04,101.09 90.04,98.04 89.79,97.79 89.79,95.38 89.98,95.19 90.3,94.87 90.72,94.45 U1.40
GPIO5
  Top 0.254: U1.43 87.72,95.54 79.53,103.72 75.4,103.72 74.3,102.62 J15.2
GPIO6
  Top 0.254: U1.44 86.72,95.74 81.24,101.22 75.31,101.22 74.3,100.2 J15.3
GPIO7
  Top 0.254: U1.45 85.72,95.9 82.94,98.68 75.56,98.68 J15.4
HBT_RX
  Top 0.305: U6.2 107.98,91.41 106.93,92.46 WIFI_RX.6
  Top 0.61: D4.2 101.71,94.11 WIFI_RX.8 WIFI_RX.7 WIFI_RX.6 WIFI_RX.5 WIFI_RX.4 WIFI_RX.3 WIFI_RX.2 WIFI_RX.1
HBT_TX
  Top 0.406: D2.2 98.81,99.19 97.79,98.17 97.79,96.14 101.22,92.71 104.39,92.71 105.38,91.72 105.38,91.66 U6.6
  Top 0.61: WIFI_TX.8 D2.2
  Bottom 0.61: WIFI_TX.8 WIFI_TX.7 WIFI_TX.6 WIFI_TX.5 WIFI_TX.4 WIFI_TX.3 WIFI_TX.2 WIFI_TX.1
MISO
  Top 0.203: R20.1 116.46,85.47 112.14,81.15 112.14,78.36 R5.1
  Top 0.305: R20.1 121.28,84.45 132.59,84.45 U2.38
MOSI
  Top 0.305: U5.2 117.5,88.29 117.8,88.58 121.35,88.58 121.92,88.01 R4.2 122.05,86.87 132.46,86.87 133.48,87.88 135.51,87.88 135.89,87.5 135.89,85.22 U2.34
N$1
  Top 0.305: R10.1 133.35,90.93 136.78,87.5 136.78,86.87 U2.33
N$2
  Top 0.254: BOOT.1 88.77,95.5 89.72,94.56 U1.41
N$3
  Top 0.203: R4.1 121.16,86.23 119.63,86.23 119.38,85.98 116.33,85.98 110.99,80.63 108.47,80.63 107.95,81.15 107.95,82.4 U3.2
N$4  (via drill 0.3 pad 0.64)
  Top 0.254: U3.12 107.33,79.01 107.95,79.63 v111.38,79.63 | v117.09,79.63 119.89,79.63 121.79,81.53 121.79,81.66 R6.1
  Bottom 0.305: v111.38,79.63 111.72,79.29 116.76,79.29 v117.09,79.63
N$6  (via drill 0.3 pad 0.64)
  Top 0.203: v104.65,77.85 104.65,76.61 U3.8 | R5.2 111.25,77.47 108.97,77.47 v108.59,77.85
  Bottom 0.203: v104.65,77.85 v108.59,77.85
N$7  (via drill 0.3 pad 0.61)
  Top 0.254: FUNCTION.1 73.66,66.93 75.82,64.77 R9.1 80.52,64.77 83.06,67.31 v84.96,67.31 | v88.65,94.23 88.65,92.88 U1.42
  Bottom 0.254: v88.65,94.23 88.65,91.44 86.74,89.53 86.74,69.09 v84.96,67.31
N$8
  Top 0.61: U4.3 112.33,65.47 111.25,64.39 109.8,64.39 L1.1
  pour Top (isolate 0.254, no thermals): 107.76,65.85 113.27,65.85 arc-90 113.41,65.71 113.41,65.28 arc-90 113.03,64.9 112.52,64.9 arc90 112.14,64.52 112.14,63.88 arc-90 111.76,63.5 107.76,63.5 arc-90 107.38,63.88 107.38,65.47 arc-90
N$9
  Top 0.406: R17.2 WRST.+
N$10
  Top 1.016: L2.1 111,67.94 110.49,67.44 109.73,67.44 109.6,67.56 109.68,67.56 L1.2
  pour Top (isolate 0.254, no thermals): 110.24,68.71 110.24,69.47 arc-90 110.62,69.85 111.51,69.85 arc-90 111.89,69.47 111.89,66.93 arc-90 111.51,66.55 107.76,66.55 arc-90 107.38,66.93 107.38,67.94 arc-90 107.76,68.33 109.86,68.33 arc90
N$12  (via drill 0.3 pad 0.61)
  Top 0.254: MODE.- 84.46,60.58 v83.57,61.47 | U1.49 84.31,90.31 v84.33,90.3
  Bottom 0.254: 83.57,61.59 v83.57,61.47 83.44,61.59 83.44,89.41 v84.33,90.3
N$13  (via drill 0.3 pad 0.61)
  Top 0.254: U1.48 v84.33,91.31 | v82.55,63.63 81.15,63.63 WIFI.-
  Bottom 0.254: v84.33,91.31 84.07,91.31 83.63,90.87 83.31,90.55 82.93,90.17 82.93,64.01 v82.55,63.63
N$15
  Top 0.406: WIFI.+ R16.1
N$18
  Top 0.406: R15.1 MODE.+
N$20  (via drill 0.3 pad 0.64)
  Top 0.254: U1.34 96.72,94.04 v96.65,94.11
  Top 0.406: 94.87,61.47 94.36,61.47 | 94.36,61.47 v89.28,61.47 88.65,60.83 SW1.1 | WRST.- 94.62,61.72 | 94.62,61.72 94.36,61.47 | 94.62,61.72 94.87,61.47 | 94.87,61.47 96.01,61.47 D3.+
  Bottom 0.254: P1.1 87.88,62.86 87.38,63.37 87.38,89.28 91.06,92.96 95.5,92.96 v96.65,94.11
  Bottom 0.406: P1.1 88.65,62.1 v89.28,61.47
N$23
  Top 0.61: Q3.1 93.22,70.23 R2.2 R11.2
N$24  (via drill 0.3 pad 0.64)
  Top 0.203: 116.84,87.52 U5.3
  Top 0.254: R18.2 113.03,78.74 113.03,80.9 v113.41,81.28 | 116.84,87.52 116.84,88.46 v117.73,89.34
  Bottom 0.254: v113.41,81.28 116.59,81.28 117.73,82.42 v117.73,89.34
N$26
  Top 0.406: R7.2 PWR.-
N$27
  Top 0.254: U3.5 106.03,83.17 106.3,83.44 110.24,83.44 R8.1
N$28
  Top 0.305: U5.8 114.21,79.09 R19.2
N$29
  Top 0.203: U5.6 114.91,86.77 115.22,86.45 119.09,86.45 119.63,87 R20.2
N$30  (via drill 0.3 pad 0.64)
  Top 0.254: U5.4 v116.21,88.9 | U5.11 116.21,83.06 v115.95,83.31
  Top 0.305: U5.11 116.21,78.61 R21.2
  Bottom 0.254: v115.95,83.31 115.95,88.65 v116.21,88.9
N$39
  Top 0.254: C18.1 R1.1 R3.1 115.95,67.69 115.63,67.37 U4.5
RESET
  Top 0.305: D3.- 99.44,64.26 104.14,59.56 U2.30 105.41,57.28 118.49,57.28 121.03,59.82 124.58,59.82 127.38,62.61 127.38,80.64 128.14,81.41 U2.36
SCK
  Top 0.203: R6.2 121.67,83.31 120.78,84.2 115.85,84.2 114.94,83.28 114.94,81.69 U5.9
  Top 0.305: R6.2 133.99,83.31 U2.37
SD_CS
  Top 0.254: R21.1 116.59,75.15 118.46,73.28 J6.2
SD_MISO  (via drill 0.3 pad 0.64)
  Top 0.254: U5.5 115.56,88.53 115.44,88.65 115.44,89.29 116.22,90.06 122.41,90.06 v124.08,88.39
  Top 0.305: J6.7 123.02,67.78 124.08,68.83 v124.08,81.91
  Bottom 0.305: v124.08,81.91 v124.08,88.39
SD_MOSI
  Top 0.254: J6.3 121.24,72.14 118.87,72.14 115.95,75.06 115.19,75.06 R18.1
SD_SCK
  Top 0.203: R19.1 115.82,77.47 122.17,77.47 123.44,76.2 123.44,70.61 122.81,69.98 J6.5
VCC_3V3  (via drill 0.3 pad 0.61, 0.3 pad 0.64)
  Top 0.406: U5.14 118.36,81.66 | U6.14 108.84,84.58 | 108.84,76.71 108.81,76.71 U3.14 | R15.2 R16.2 v79.63,60.58
  Top 0.61: U1.3 85.72,73.03 86.11,72.64 C2.2 | C19.2 C20.2 110.11,84.58 v109.6,84.58 | C22.2 121.2,70.99 J6.4 | 118.36,81.66 120.14,81.66 C23.2 v120.27,81.03 | C1.2 108.84,76.71 | 101.22,88.27 107.44,88.27 108.84,86.87 108.84,84.58 v109.6,84.58 | 101.22,88.27 100.71,88.77 | 101.22,88.27 100.71,87.76 | U1.2 84.72,72.02 84.71,72.01 | U1.5 87.72,72.1 C4.2 | U1.27 99.52,86.31 100.08,86.87 C7.2 C12.2 100.68,85.31 U1.26 | v109.6,84.58 | U1.38 92.72,94.62 C6.2 C5.2 91.31,95.25 v90.55,96.01 | v84.46,96.01 81.41,96.01 80.01,97.41 J14.4 | Q3.2 90.93,69.72 90.93,64.26 PWR.+ 91.31,64.01 v92.2,63.12 92.84,62.48 R17.1
  Top 0.813: C6.2 97.41,95.25 100.71,91.95 100.71,88.77 100.71,87.76 C7.2 | C24.+ C11.2 C9.2 108.84,70.99 C10.2 L2.2 111.12,70.99 C18.2 R1.2 | C22.2 C21.2 117.6,72.26 115.95,73.91 111,73.91 | C1.2 v110.49,75.82 110.49,74.42 | 110.49,74.42 110.49,73.91 | 110.49,73.91 111,73.91 | 109.98,73.91 105.28,73.91 103.63,72.26 C24.+ | 109.98,73.91 110.49,73.91 | 90.68,72.01 C4.2 C2.2 84.71,72.01 C3.2 83.82,72.01 83.31,71.5 83.31,68.83 80.77,66.29 v80.14,66.29 R9.2 | 90.68,72.01 91.19,72.01 | 91.19,72.01 91.69,72.01 | 91.69,72.01 98.68,72.01 99.7,70.99 C24.+ | Q3.2 91.19,71.5 | 91.19,71.5 91.19,72.01 | 91.19,71.5 90.68,72.01 | 91.19,71.5 91.69,72.01 | 110.49,74.42 109.98,73.91 | 110.49,74.42 111,73.91
  Bottom 0.406: v79.63,60.58 79.63,65.79 v80.14,66.29
  Bottom 0.61: 110.49,78.99 110.49,78.36 | 110.49,78.36 v110.49,75.82 | 110.87,78.61 117.86,78.61 118.75,79.5 118.75,80.64 | 110.87,78.61 110.74,78.61 110.49,78.36 | 110.87,78.61 110.49,78.99 | 118.75,81.03 118.75,81.41 119.13,81.03 | 118.75,81.03 118.75,80.64 | v120.27,81.03 119.13,81.03 | 119.13,81.03 118.75,81.03 | 119.13,81.03 118.75,80.64 | 110.49,78.99 110.49,83.69 v109.6,84.58 | v90.55,96.01 v84.46,96.01 | 3V3.T 92.33,62.99 v92.2,63.12
VCC_5V  (via drill 0.3 pad 0.64)
  Top 0.254: U4.1 114.29,67.37 114.49,67.17 114.49,65.67 114.7,65.47 U4.4
  Top 0.813: U4.4 116.91,65.47 | 116.91,65.47 C17.2 | 116.91,65.47 118.94,65.47 C8.2 119,61.34 | 119,61.34 119,60.71 119.13,60.58 | 119,61.34 118.36,60.71 | 119,61.34 119.63,60.71 | C16.2 C13.2 126.87,92.33 125.86,91.31 125.86,88.52 v125.98,88.39 | C16.2 C15.2 C14.2 R10.2 133.35,93.22 132.33,94.23 132.33,96.9 132.84,97.41 133.84,97.41 SERIAL.3 | I2C.3 127.75,97.55 128.65,96.65 128.65,92.46 C16.2
  Top 1.016: 109.73,60.58 106.68,60.58 99.95,67.31 97.54,67.31 R11.1 | 109.73,60.58 119.13,60.58 119.51,60.96 124.33,60.96 125.98,62.61 v125.98,81.41 | 109.73,60.58 109.22,60.07 U2.28
  Bottom 1.016: v125.98,81.41 v125.98,88.39
VCC_M_3V3
  Top 1.016: Q3.3 94.23,65.79 99.44,65.79 U2.29
W_CS  (via drill 0.3 pad 0.64)
  Top 0.203: U3.10 106.03,78.75 v105.41,79.38
  Top 0.254: U1.24 101.98,83.31 103.89,81.41 v105.41,81.41 105.41,82.4 U3.6
  Bottom 0.203: v105.41,79.38 v105.41,81.41
W_MISO
  Top 0.254: U3.9 105.38,78.13 104.27,79.25 103.5,79.25 102.49,80.26 98.77,80.26 U1.21
W_MOSI
  Top 0.254: U1.23 102.22,82.31 103.9,80.63 107.02,80.63 107.31,80.93 107.31,82.41 U3.3
W_SCK
  Top 0.254: U1.22 102.46,81.31 103.63,80.14 106.32,80.14 106.68,79.78 U3.11
WIFI_CTS  (via drill 0.3 pad 0.61)
  Top 0.254: U1.62 83.85,77.31 85.44,77.31 v85.6,77.47
  Bottom 0.254: v85.6,77.47 85.6,78.23 86.23,78.87 86.23,92.58 82.68,96.14 82.68,99.19 J14.1
WIFI_RTS  (via drill 0.3 pad 0.61)
  Top 0.254: U1.61 84.25,78.31 v84.46,78.1
  Bottom 0.254: v84.46,78.1 84.58,78.1 85.7,79.22 85.7,92.23 81.79,96.14 81.79,96.9 77.09,101.6 77.09,102.23 J14.2
WIFI_RX  (via drill 0.3 pad 0.64)
  Top 0.254: 107.31,90.41 U6.3 | U1.63 87.74,76.31 v88.77,77.34
  Top 0.305: v106.17,91.69 106.93,91.69 107.33,91.3 U6.3
  Bottom 0.305: v106.17,91.69 91.82,77.34 v88.77,77.34
WIFI_S_CLK  (via drill 0.3 pad 0.61)
  Top 0.254: v84.58,79.12 84.07,79.12 83.95,79.25 82.98,79.25 U1.60
  Bottom 0.254: v84.58,79.12 85.15,79.69 85.15,91.63 J14.3
WIFI_TX  (via drill 0.3 pad 0.64)
  Top 0.254: 106.05,90.41 U6.5 | U1.64 83.82,75.31 84.33,75.82 88.27,75.82 v88.77,76.33
  Top 0.305: U6.5 106.03,89.3 v106.05,89.28
  Bottom 0.305: v106.05,89.28 104.65,89.28 91.69,76.33 v88.77,76.33

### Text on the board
tPlace: IO1 | W_CTS | IO5 | W_RTS | D7 | D0 | A5 | D9 | A4 | IO6 | W_CLK | D8 | IO7 | 3V3 | VCC | VCC | GND | GND | GND | GND | D7 | D0
bPlace: Wifi Shield(FI250) | v1.11 12/15/2014 | by Seeed Studio | www.seeedstudio.com

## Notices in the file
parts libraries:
moudle-new: This work is licensed under the Creative Commons Attribution 4.0 International License.
To view a copy of this license,visit:
http://creativecommons.org/licenses/by-sa/4.0
moudle-new: CC-BY-SA
